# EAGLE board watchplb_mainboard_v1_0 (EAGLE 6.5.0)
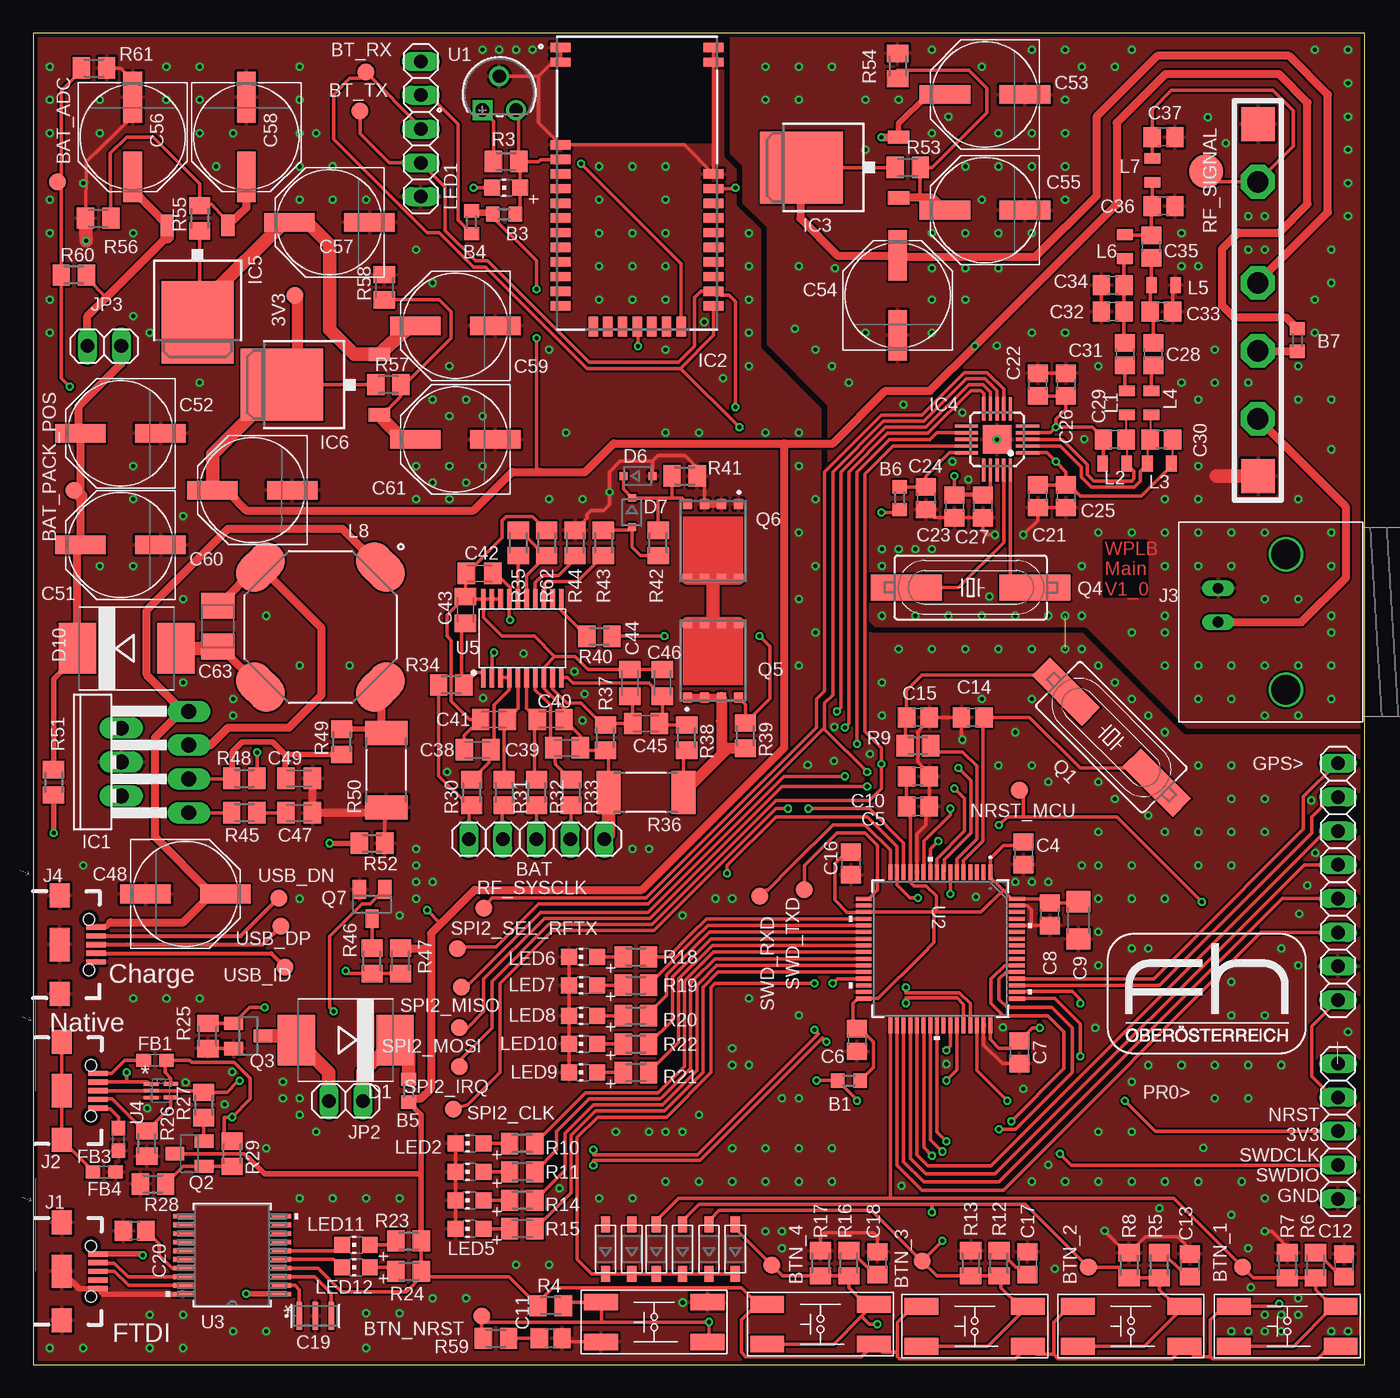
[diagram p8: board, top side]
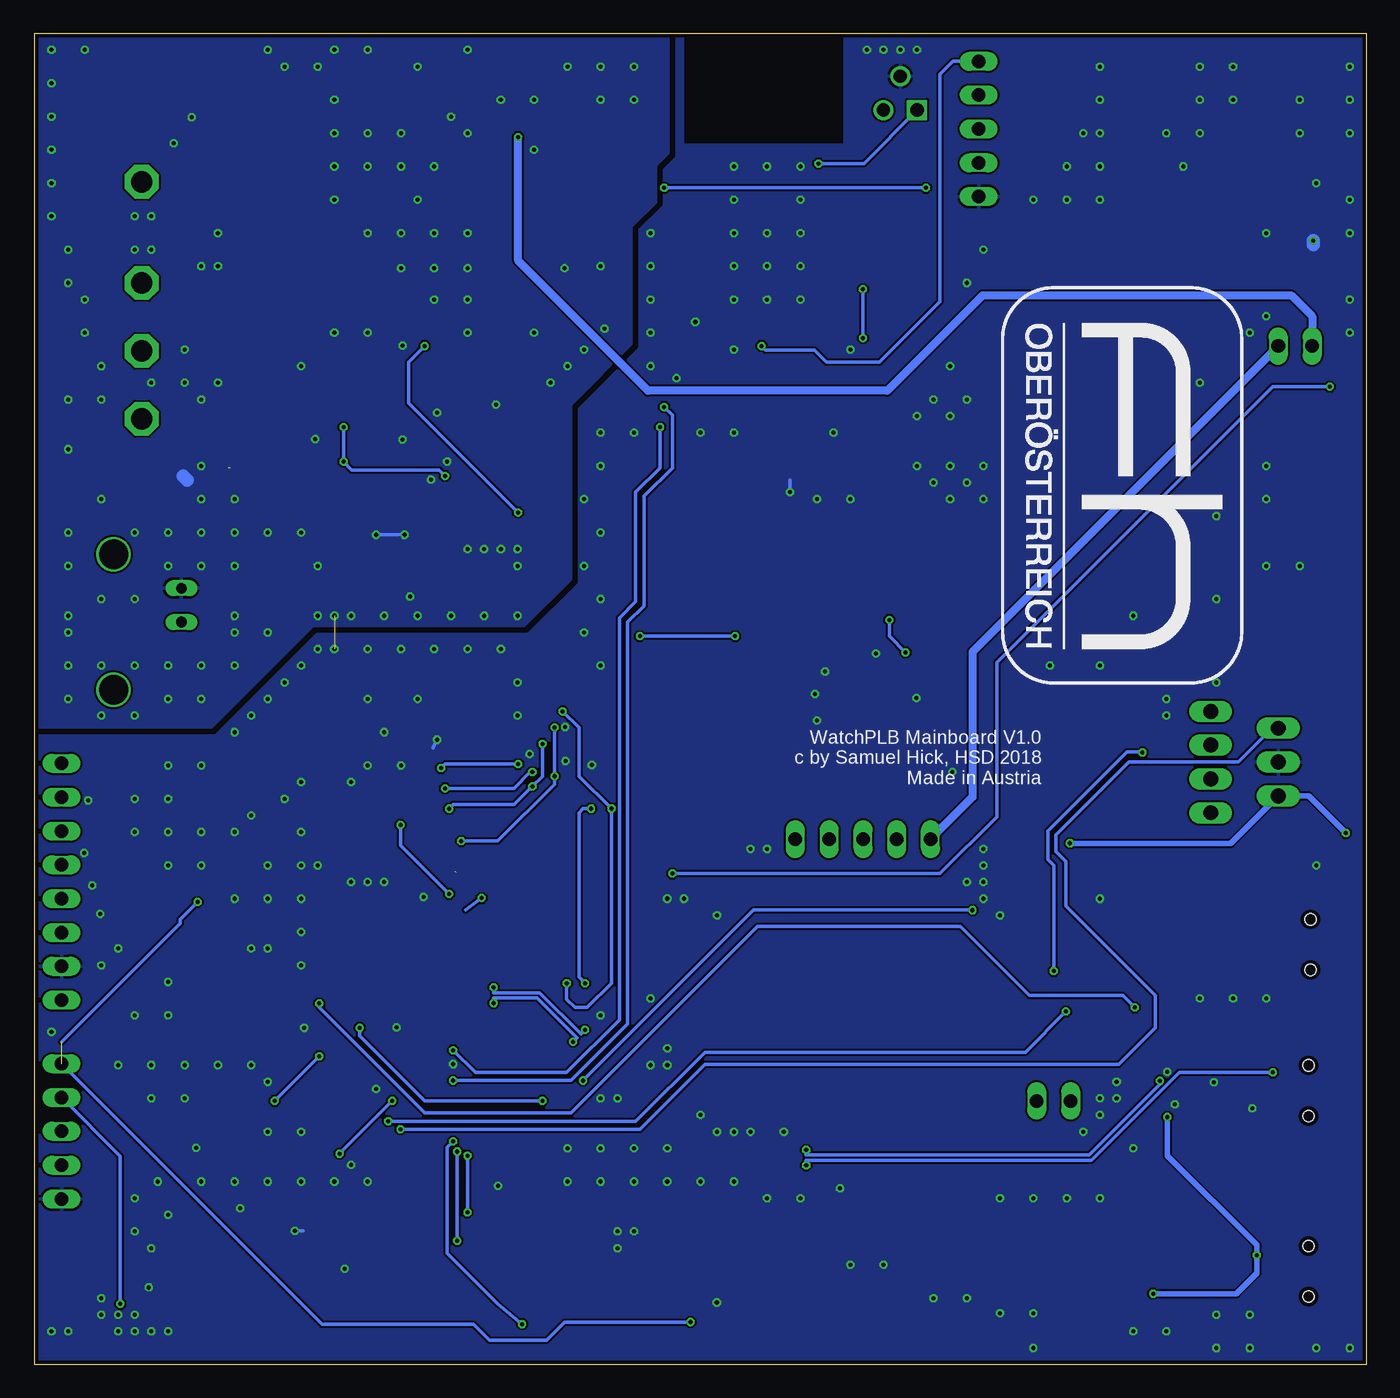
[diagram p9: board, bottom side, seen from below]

Size 100 x 100 mm. Coordinates in mm from the lower left corner, seen from the top.
Outline: 0,0 100,0 100,100 0,100 0,0
Copper layers (1*16): Top 0.035mm / dielectric 1.5mm / Bottom 0.035mm
Design rules "PCB-POOL Standard": minimum track width 0.15mm, minimum drill 0.3mm, track to track 0.15mm, track to pad 0.15mm, pad to pad 0.15mm, via to via 0.15mm, smd to smd 0.15mm, copper to edge 0.3mm, drill to drill 0.2mm, minimum pad ring 0.2mm, minimum via ring 0.15mm, stop-mask expansion 0.075mm, vias tented up to drill 0mil, thermal gap 0.2mm
tRestrict: area 39.3,91.7 to 51.2,99.7; 11 lines
bRestrict: area 39.3,91.7 to 51.2,99.7; 11 lines

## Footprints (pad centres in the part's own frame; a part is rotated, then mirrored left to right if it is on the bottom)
B1,27 = smd 1.27 x 1.27: TP 0,0
L0603 = smd 1 x 1.1: 1 -0.85,0; 2 0.85,0
1X05 = drill 1.016 long: 1 -5.08,0; 2 -2.54,0; 3 0,0; 4 2.54,0; 5 5.08,0
C0805 = smd 1.3 x 1.5: 1 -0.85,0; 2 0.85,0
C1206 = smd 1.6 x 1.8: 1 -1.4,0; 2 1.4,0
CSTCE = smd 0.406 x 2.108: 1 -1.2,0; 2 0,0; 3 1.2,0
C0805K = smd 1.3 x 1.6: 1 -1,0; 2 1,0
PANASONIC_E = smd 3.8 x 1.4: + 3,0; - -3,0
B/3528-21R = smd 1.95 x 2.5: + 1.525,0; - -1.525,0
SMC = smd 2.8 x 3.8: A 3.7,0; C -3.7,0
SOD-123 = smd 1.2 x 0.7: A 1.85,0; C -1.85,0
SOD323-R = smd 0.6 x 0.6: A 1.1,0; C -1.1,0
0603 = smd 1.1 x 1: 1 -0.85,0; 2 0.85,0
1X08 = drill 1.016 long: 1 -8.89,0; 2 -6.35,0; 3 -3.81,0; 4 -1.27,0; 5 1.27,0; 6 3.81,0; 7 6.35,0; 8 8.89,0
TO220-7 = drill 1.118 pad 1.626 long: 1 -3.81,-8.636; 2 -2.54,-3.556; 3 -1.27,-8.636; 4 0,-3.556; 5 1.27,-8.636; 6 2.54,-3.556; 7 3.81,-8.636
BM78SPPS5NC2_1 = smd 1.5 x 0.7: 1 -11.75,21.2; 2 -11.75,20.1; 3 -11.75,13.9; 4 -11.75,12.8; 5 -11.75,11.7; 6 -11.75,10.6; 7 -11.75,9.5; 8 -11.75,8.4; 9 -11.75,7.3; 10 -11.75,6.2; 11 -11.75,5.1; 12 -11.75,4; 13 -11.75,2.9; 14 -11.75,1.8; 22 -0.25,1.8; 23 -0.25,2.9; 24 -0.25,4; 25 -0.25,5.1; 26 -0.25,6.2; 27 -0.25,7.3; 28 -0.25,8.4; 29 -0.25,9.5; 30 -0.25,10.6; 31 -0.25,11.7; 32 -0.25,20.1; 33 -0.25,21.2 | smd 0.7 x 1.5: 15 -9.3,0.25; 16 -8.2,0.25; 17 -7.1,0.25; 18 -6,0.25; 19 -4.9,0.25; 20 -3.8,0.25; 21 -2.7,0.25
TO252 = smd 1 x 1.6: 1 -2.28,-4.8; 2 2.28,-4.8 | smd 5.4 x 6.2: TAB 0,2.5
QFN20 = smd 0.25 x 1.75: 1 -1,-2.3; 2 -0.5,-2.3; 3 0,-2.3; 4 0.5,-2.3; 5 1,-2.3; 11 1,2.3; 12 0.5,2.3; 13 0,2.3; 14 -0.5,2.3; 15 -1,2.3 | smd 1.75 x 0.25: 6 2.3,-1; 7 2.3,-0.5; 8 2.3,0; 9 2.3,0.5; 10 2.3,1; 16 -2.3,1; 17 -2.3,0.5; 18 -2.3,0; 19 -2.3,-0.5; 20 -2.3,-1 | smd 2.15 x 2.15: PAD 0,0
USB-B-MICRO-SMD = smd 1.45 x 0.4: D+ 2.725,0; D- 2.725,0.65; GND 2.725,-1.3; ID 2.725,-0.65; VBUS 2.725,1.3 | smd 1.5 x 1.8: SHIELD1 0,3.685; SHIELD2 0,-3.685 | smd 1.5 x 2.5: SHIELD3 0,0 | hole 0.85: 2.2,1.9; 2.2,-1.9
BNC = drill 2.2: 3 -5.08,5.08; 4 5.08,5.08 | drill 0.8 long: GND -2.54,0; S 0,0
1X02 = drill 1.016 long: 1 -1.27,0; 2 1.27,0
0805 = smd 0.8 x 1.2: 1 -0.9,0; 2 0.9,0
INDM115115X635N = smd 2.769 x 4.064: 1 -6.375,0; 3 6.375,0 | smd 4.064 x 2.769: 2 0,-6.375; 4 0,6.375
CHIP-LED0805 = smd 1.2 x 1.2: A 0,-1.05; C 0,1.05
HC49UP = smd 5.334 x 1.93: 1 -4.826,0; 2 4.826,0
SOT23-BEC = smd 1 x 1.4: B -0.95,-1.1; C 0,1.1; E 0.95,-1.1
SOT23 = smd 1 x 1.4: 1 -0.95,-1.1; 2 0.95,-1.1; 3 0,1.1
TRANS_CSD18534Q5A = smd 0.75 x 0.68: 1 -2.77,1.905; 2 -2.77,0.635; 3 -2.77,-0.635; 4 -2.77,-1.905 | smd 0.66 x 0.68: 5 2.78,-1.905; 6 2.78,-0.635; 7 2.78,0.635; 8 2.78,1.905
M0805 = smd 1.3 x 1.6: 1 -0.95,0; 2 0.95,0
R2512 = smd 1.8 x 3.2: 1 -2.8,0; 2 2.8,0
B2,54 = smd 2.54 x 2.54: TP 0,0
SMD_SWITCH = smd 2.54 x 1.27: P$1 4,1.5; P$2 -4,-1.5; P$3 -4,1.5; P$4 4,-1.5
TO-92_MC = drill 0.991 pad 1.499 square: 1 -2.54,-2.54 | drill 0.991 pad 1.499: 2 -1.27,0; 3 0,-2.54
LQFP64-10X10MM = smd 1.194 x 0.305: 1 -5.75,3.75; 2 -5.75,3.25; 3 -5.75,2.75; 4 -5.75,2.25; 5 -5.75,1.75; 6 -5.75,1.25; 7 -5.75,0.75; 8 -5.75,0.25; 9 -5.75,-0.25; 10 -5.75,-0.75; 11 -5.75,-1.25; 12 -5.75,-1.75; 13 -5.75,-2.25; 14 -5.75,-2.75; 15 -5.75,-3.25; 16 -5.75,-3.75; 33 5.75,-3.75; 34 5.75,-3.25; 35 5.75,-2.75; 36 5.75,-2.25; 37 5.75,-1.75; 38 5.75,-1.25; 39 5.75,-0.75; 40 5.75,-0.25; 41 5.75,0.25; 42 5.75,0.75; 43 5.75,1.25; 44 5.75,1.75; 45 5.75,2.25; 46 5.75,2.75; 47 5.75,3.25; 48 5.75,3.75 | smd 0.305 x 1.194: 17 -3.75,-5.75; 18 -3.25,-5.75; 19 -2.75,-5.75; 20 -2.25,-5.75; 21 -1.75,-5.75; 22 -1.25,-5.75; 23 -0.75,-5.75; 24 -0.25,-5.75; 25 0.25,-5.75; 26 0.75,-5.75; 27 1.25,-5.75; 28 1.75,-5.75; 29 2.25,-5.75; 30 2.75,-5.75; 31 3.25,-5.75; 32 3.75,-5.75; 49 3.75,5.75; 50 3.25,5.75; 51 2.75,5.75; 52 2.25,5.75; 53 1.75,5.75; 54 1.25,5.75; 55 0.75,5.75; 56 0.25,5.75; 57 -0.25,5.75; 58 -0.75,5.75; 59 -1.25,5.75; 60 -1.75,5.75; 61 -2.25,5.75; 62 -2.75,5.75; 63 -3.25,5.75; 64 -3.75,5.75
SSOP20_MC = smd 1.473 x 0.356: 1 -3.708,2.926; 2 -3.708,2.276; 3 -3.708,1.626; 4 -3.708,0.975; 5 -3.708,0.325; 6 -3.708,-0.325; 7 -3.708,-0.975; 8 -3.708,-1.626; 9 -3.708,-2.276; 10 -3.708,-2.926; 11 3.708,-2.926; 12 3.708,-2.276; 13 3.708,-1.626; 14 3.708,-0.975; 15 3.708,-0.325; 16 3.708,0.325; 17 3.708,0.975; 18 3.708,1.626; 19 3.708,2.276; 20 3.708,2.926
SOT50P160X60-5N = smd 1.118 x 0.254: 1 -0.737,0.508; 2 -0.737,0; 3 -0.737,-0.508 | smd 1.118 x 0.305: 4 0.737,-0.508; 5 0.737,0.508
TSSOP-20/6MM = smd 1.5 x 0.35: 1 -2.95,2.925; 2 -2.95,2.275; 3 -2.95,1.625; 4 -2.95,0.975; 5 -2.95,0.325; 6 -2.95,-0.325; 7 -2.95,-0.975; 8 -2.95,-1.625; 9 -2.95,-2.275; 10 -2.95,-2.925; 11 2.95,-2.925; 12 2.95,-2.275; 13 2.95,-1.625; 14 2.95,-0.975; 15 2.95,-0.325; 16 2.95,0.325; 17 2.95,0.975; 18 2.95,1.625; 19 2.95,2.275; 20 2.95,2.925
RA07H4047M = drill 1.6 pad 2.54 octagon: 1 6.1,1.75; 2 13.7,1.75; 3 18.8,1.75; 4 23.9,1.75 | smd 2.54 x 2.54: 5_L 1.778,1.778; 5_R 28.194,1.778

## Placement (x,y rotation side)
3V3  PTR1B1,27  [B1,27]  19.66,80.31 90 top
B1  BLM18KG601SN1D  [L0603]  61.26,21.34 0 top
B3  BLM18KG601SN1D  [L0603]  35.36,86.41 0 top
B4  BLM18KG601SN1D  [L0603]  32.92,85.8 270 top
B5  BLM18KG601SN1D  [L0603]  28.19,20.57 90 top
B6  BLM18KG601SN1D  [L0603]  65.07,65.07 90 top
B7  BLM18KG601SN1D  [L0603]  94.95,76.96 270 top
BAT  [1X05]  37.8,39.47 0 top
BAT_ADC  PTR1B1,27  [B1,27]  1.83,88.85 0 top
BAT_PACK_POS  PTR1B1,27  [B1,27]  3.05,65.68 0 top
BT_RX  PTR1B1,27  [B1,27]  24.99,97.08 0 top
BT_TX  PTR1B1,27  [B1,27]  24.54,94.18 0 top
BTN_1  PTR1B1,27  [B1,27]  90.83,7.32 180 top
BTN_2  PTR1B1,27  [B1,27]  79.25,7.32 180 top
BTN_3  PTR1B1,27  [B1,27]  66.75,7.77 180 top
BTN_4  PTR1B1,27  [B1,27]  55.47,7.47 180 top
BTN_NRST  PTR1B1,27  [B1,27]  33.68,3.66 180 top
C4  100nF  [C0805]  74.37,38.4 270 top
C5  100nF  [C0805]  66.45,41.91 180 top
C6  100nF  [C0805]  61.87,24.38 90 top
C7  100nF  [C0805]  74.07,23.47 270 top
C8  100nF  [C0805]  76.35,33.83 270 top
C9  10uF  [C1206]  78.49,33.38 270 top
C10  1uF  [C0805]  66.45,44.2 180 top
C11  100nF  [C0805]  38.86,1.98 180 top
C12  100nF  [C0805]  98.45,7.47 270 top
C13  100nF  [C0805]  86.87,7.47 270 top
C14  27p  [C0805]  70.56,48.62 180 top
C15  27p  [C0805]  66.45,48.62 0 top
C16  100nF  [C0805]  61.42,37.64 90 top
C17  100nF  [C0805]  74.68,7.62 270 top
C18  100nF  [C0805]  63.4,7.62 270 top
C19  CSTCE12M0G15L99-R0  [CSTCE]  21.18,3.66 0 top
C20  1uF  [C0805]  7.62,10.06 180 top
C21  100nF  [C0805]  75.44,65.23 90 top
C22  100nF  [C0805]  75.44,73.61 270 top
C23  100nF  [C0805]  69.19,64.47 90 top
C24  100nF  [C0805]  67.06,65.07 90 top
C25  27pF  [C0805]  77.57,65.23 90 top
C26  27pF  [C0805]  77.57,73.61 270 top
C27  1uF  [C0805]  71.32,64.47 90 top
C28  [C0805]  84.12,75.9 90 top
C29  [C0805]  81.23,69.49 180 top
C30  [C0805]  84.73,69.49 180 top
C31  [C0805]  81.99,75.9 90 top
C32  [C0805]  81.08,79.1 0 top
C33  [C0805]  84.73,79.1 0 top
C34  [C0805]  81.08,81.08 0 top
C35  [C0805]  83.97,83.97 270 top
C36  [C0805]  84.89,87.02 180 top
C37  [C0805]  84.89,92.2 180 top
C38  100nF  [C0805K]  33.38,46.18 180 top
C39  100nF  [C0805K]  40.08,46.33 0 top
C40  100nF  [C0805K]  38.86,48.46 0 top
C41  100nF  [C0805K]  34.59,48.46 180 top
C42  1uF  [C0805K]  33.53,59.44 0 top
C43  1uF  [C0805K]  32.46,56.69 90 top
C44  100nF  [C0805K]  44.81,51.21 270 top
C45  100nF  [C0805K]  46.02,48.16 0 top
C46  100nF  [C0805K]  47.24,51.21 90 top
C47  100nF  [C0805K]  19.96,41.45 180 top
C48  22uF 80-EDK226M050A9GAA  [PANASONIC_E]  11.43,35.36 0 top
C49  100nF  [C0805K]  19.96,44.04 180 top
C51  22uF 80-EDK226M050A9GAA  [PANASONIC_E]  6.55,61.57 180 top
C52  22uF 80-EDK226M050A9GAA  [PANASONIC_E]  6.55,69.95 180 top
C53  10uF 80-EDK106M025A9DAA  [PANASONIC_E]  71.48,95.4 180 top
C54  100uF 647-GYA1E101MCQ1GS  [PANASONIC_E]  64.92,80.31 90 top
C55  NP  [PANASONIC_E]  71.48,86.72 180 top
C56  10uF 80-EDK106M025A9DAA  [PANASONIC_E]  7.47,92.2 270 top
C57  100uF 647-GYA1E101MCQ1GS  [PANASONIC_E]  22.25,85.8 180 top
C58  NP  [PANASONIC_E]  16,92.2 270 top
C59  10uF 80-EDK106M025A9DAA  [PANASONIC_E]  31.7,78.03 180 top
C60  100uF 647-GYA1E101MCQ1GS  [PANASONIC_E]  16.46,65.68 180 top
C61  NP  [PANASONIC_E]  31.7,69.49 180 top
C63  4.7uF low esr 80-T521B475M35ATE150  [B/3528-21R]  13.87,55.47 90 top
CONFIG_INTERFACE_TEST_POINT  [1X05]  29.11,92.81 270 top
D1  S8NC-13  [SMC]  23.47,24.38 180 top
D2  [SOD-123]  46.79,8.69 90 top
D3  [SOD-123]  48.77,8.69 90 top
D4  [SOD-123]  50.75,8.69 90 top
D5  [SOD-123]  52.73,8.69 90 top
D6  Zener 16V MMSZ5246BS-7-F  [SOD323-R]  45.42,66.75 0 top
D7  100V, BAS16J,135  [SOD323-R]  44.96,64.01 270 top
D8  [SOD-123]  44.96,8.69 90 top
D9  [SOD-123]  42.98,8.69 90 top
D10  MBRS330T3  [SMC]  7.01,53.8 0 top
FB1  BLM18PG300SN1D  [0603]  9.14,22.86 0 top
FB3  BLM18PG300SN1D  [0603]  6.4,16.92 90 top
FB4  BLM18PG300SN1D  [0603]  5.33,14.48 180 top
GPS>  [1X08]  97.99,36.27 90 top
IC1  LT1513  [TO220-7]  3.05,45.26 90 top
IC2  BM70BLES1FC2-0B03AA  [BM78SPPS5NC2_1]  51.36,77.72 0 top
IC3  LM1117DTX-ADJ-12V  [TO252]  60.2,89.92 90 top
IC4  AX5031  [QFN20]  72.39,69.49 90 top
IC5  LM1117DTX-ADJ-10V  [TO252]  12.34,80.77 180 top
IC6  LM1117DTX-ADJ-3V3  [TO252]  21.18,73.61 90 top
J1  [USB-B-MICRO-SMD]  2.13,7.01 0 top
J2  [USB-B-MICRO-SMD]  2.13,20.57 0 top
J3  BNCPTH  [BNC]  89,55.78 270 top
J4  [USB-B-MICRO-SMD]  1.98,31.55 0 top
JP2  VIB_MOTOR, 619-28821  [1X02]  23.47,19.81 180 top
JP3  Power Disconnect  [1X02]  5.33,76.5 180 top
L1  [0805]  82.14,72.24 270 top
L2  [0805]  81.23,67.67 0 top
L3  [0805]  84.58,67.67 0 top
L4  [0805]  83.97,72.24 270 top
L5  [0805]  84.89,81.08 180 top
L6  [0805]  81.99,83.97 90 top
L7  [0805]  84.05,89.69 90 top
L8  CTX10-4A-R  [INDM115115X635N]  21.57,55.4 225 top
LED1  BLUE  [CHIP-LED0805]  35.51,88.39 90 top
LED2  GREEN  [CHIP-LED0805]  32.77,16.61 90 top
LED3  BLUE  [CHIP-LED0805]  32.77,14.48 90 top
LED4  WHITE  [CHIP-LED0805]  32.77,12.34 90 top
LED5  RED  [CHIP-LED0805]  32.77,10.21 90 top
LED6  GREEN  [CHIP-LED0805]  41.3,30.63 90 top
LED7  GREEN  [CHIP-LED0805]  41.3,28.5 90 top
LED8  GREEN  [CHIP-LED0805]  41.3,26.21 90 top
LED9  RED  [CHIP-LED0805]  41.3,21.95 90 top
LED10  YELLOW  [CHIP-LED0805]  41.3,24.08 90 top
LED11  GREEN  [CHIP-LED0805]  24.23,8.99 90 top
LED12  RED  [CHIP-LED0805]  24.23,7.32 90 top
NRST_MCU  PTR1B1,27  [B1,27]  74.07,43.13 180 top
PR0>  SWD  [1X05]  97.99,17.53 90 top
Q1  8MHz / LFXTAL020423Reel  [HC49UP]  80.97,47.14 315 top
Q2  BC817-25SMD  [SOT23-BEC]  11.73,15.85 90 top
Q3  DMN3023L-7  [SOT23]  16.15,24.69 270 top
Q4  16MHz_LFXTAL051370Reel  [HC49UP]  70.41,58.37 180 top
Q5  CSD18534Q5A  [TRANS_CSD18534Q5A]  51.05,52.88 90 top
Q6  CSD18534Q5A  [TRANS_CSD18534Q5A]  51.05,61.87 270 top
Q7  DMN3023L-7  [SOT23]  25.45,34.59 180 top
R3  4k7  [M0805]  35.51,90.37 180 top
R4  47k  [M0805]  38.86,4.42 0 top
R5  10k  [M0805]  84.58,7.47 270 top
R6  10k  [M0805]  96.32,7.47 270 top
R7  10k  [M0805]  94.18,7.47 90 top
R8  10k  [M0805]  82.3,7.47 90 top
R9  220R  [M0805]  66.45,46.48 0 top
R10  470R  [M0805]  36.73,16.61 0 top
R11  470R  [M0805]  36.73,14.48 0 top
R12  10k  [M0805]  72.54,7.62 270 top
R13  10k  [M0805]  70.41,7.62 90 top
R14  470R  [M0805]  36.73,12.34 0 top
R15  470R  [M0805]  36.73,10.21 0 top
R16  10k  [M0805]  61.26,7.62 270 top
R17  10k  [M0805]  59.13,7.62 90 top
R18  470R  [M0805]  45.26,30.63 180 top
R19  470R  [M0805]  45.26,28.5 180 top
R20  470R  [M0805]  45.26,26.21 180 top
R21  470R  [M0805]  45.26,21.95 180 top
R22  470R  [M0805]  45.26,24.08 180 top
R23  220R  [M0805]  28.19,9.3 180 top
R24  220R  [M0805]  28.19,7.01 180 top
R25  100k  [M0805]  13.11,24.69 270 top
R26  100k  [M0805]  8.53,16.61 270 top
R27  x  [M0805]  12.8,19.51 90 top
R28  x  [M0805]  8.99,13.56 180 top
R29  x  [M0805]  14.94,15.85 270 top
R30  1k  [M0805]  32.92,42.98 90 top
R31  1k  [M0805]  35.36,42.98 90 top
R32  1k  [M0805]  37.8,42.98 90 top
R33  1k  [M0805]  40.39,42.98 90 top
R34  1k  [M0805]  31.39,51.05 0 top
R35  10k  [M0805]  36.42,61.72 90 top
R36  20mR  [R2512]  46.02,42.98 180 top
R37  100R  [M0805]  42.98,47.09 270 top
R38  100R  [M0805]  49.07,47.09 270 top
R39  10M  [M0805]  53.49,47.24 270 top
R40  5k1  [M0805]  42.52,54.71 180 top
R41  3M3  [M0805]  48.92,66.75 180 top
R42  1M  [M0805]  46.94,61.72 270 top
R43  5k1  [M0805]  42.82,61.72 90 top
R44  470k  [M0805]  40.69,61.72 90 top
R45  330  [M0805]  15.85,41.45 0 top
R46  910R  [M0805]  25.45,30.33 270 top
R47  10k  [M0805]  27.58,30.33 270 top
R48  330k  [M0805]  15.85,44.04 180 top
R49  10k  [M0805]  23.16,46.79 90 top
R50  0.25R  [R2512]  26.52,44.65 90 top
R51  120k  [M0805]  1.52,43.74 90 top
R52  12k4  [M0805]  25.45,39.17 180 top
R53  5k1  [M0805]  65.68,89.92 0 top
R54  47k  [M0805]  64.92,97.54 90 top
R55  5k1  [M0805]  12.5,86.11 90 top
R56  47k  [M0805]  4.88,86.11 180 top
R57  5k1  [M0805]  26.67,73.61 0 top
R58  47k  [M0805]  26.37,80.92 90 top
R59  10k  [M0805]  34.75,1.98 180 top
R60  47k  [M0805]  3.05,81.84 0 top
R61  10k  [M0805]  4.57,97.38 180 top
R62  NTC 103AT  [M0805]  38.56,61.72 90 top
RF_SIGNAL  PTR1B2,54  [B2,54]  88.09,89.61 0 top
RF_SYSCLK  PTR1B1,27  [B1,27]  33.83,34.29 180 top
S1  [SMD_SWITCH]  46.63,3.2 180 top
S2  [SMD_SWITCH]  94.18,2.9 180 top
S3  [SMD_SWITCH]  82.45,2.9 180 top
S4  [SMD_SWITCH]  70.71,2.9 180 top
S5  [SMD_SWITCH]  59.13,3.05 180 top
SPI2_CLK  PTR1B1,27  [B1,27]  31.55,19.2 180 top
SPI2_IRQ  PTR1B1,27  [B1,27]  32,22.4 180 top
SPI2_MISO  PTR1B1,27  [B1,27]  32.16,28.35 180 top
SPI2_MOSI  PTR1B1,27  [B1,27]  32,25.3 180 top
SPI2_SEL_RFTX  PTR1B1,27  [B1,27]  31.85,31.24 180 top
SWD_RXD  PTR1B1,27  [B1,27]  54.56,35.2 180 top
SWD_TXD  PTR1B1,27  [B1,27]  57.91,35.66 180 top
U1  MCP111-XXXXX/TO  [TO-92_MC]  36.27,96.77 0 top
U2  STM32L073RZ  [LQFP64-10X10MM]  68.12,31.24 270 top
U3  MCP2200-I/SS  [SSOP20_MC]  14.94,8.23 180 top
U4  TPD3E001DRLR  [SOT50P160X60-5N]  9.6,20.57 0 top
U5  BQ7790504  [TSSOP-20/6MM]  36.73,54.56 90 top
U$2  RA07H4047M  [RA07H4047M]  90.22,94.95 270 top
U$4  [FH_LOGO]  27.74,81.38 270 bottom
U$5  [FH_LOGO_050]  80.47,23.16 0 top
USB_DN  PTR1B1,27  [B1,27]  18.44,35.05 90 top
USB_DP  PTR1B1,27  [B1,27]  18.59,32.92 90 top
USB_ID  PTR1B1,27  [B1,27]  18.9,29.87 90 top

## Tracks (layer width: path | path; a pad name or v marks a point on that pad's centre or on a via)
10V_INTERMEDIATE
  Top 0.254: R55.1 12.5,78.33 IC5.TAB
  Top 0.813: C57.+ 19.4,85.65 20.73,85.65
  Top 1.016: C57.+ 18.9,85.8 13.11,80.16 13.11,78.94 IC5.TAB | C59.+ 28.35,78.03 IC6.2 24.09,75.89 22.25,77.72 22.25,84.12 20.73,85.65
+3V3  (via drill 0.3)
  Top 0.254: R57.1 19.81,73.61 IC6.TAB | 97.71,1.4 S2.P$3 98.01,1.22 97.23,1.22 96.47,0.46 88.54,0.46 88.39,0.61 | 88.39,0.61 88.39,3.35 89.31,4.27 90.06,4.27 S2.P$4 93.4,4.4 v93.57,4.57 | 76.66,0.76 76.66,3.2 77.85,4.4 S3.P$4 78.02,3.96 77.42,3.96 | S4.P$4 66.12,4.4 64.92,3.2 64.92,0.91 | 54.1,4.27 53.19,3.35 53.19,0.91 53.49,0.61 62.19,0.61 S5.P$3 63.77,0.91 64.92,0.91 | S5.P$4 54.85,4.27 54.1,4.27 | 76.66,0.76 76.96,0.46 85.51,0.46 S3.P$3 87.23,0.61 88.39,0.61 | 76.66,0.76 75.35,0.76 S4.P$3 73.78,0.46 65.08,0.46 64.92,0.61 64.92,0.91 | 54.1,4.27 54.41,4.57 | Q2.C 15.85,15.85 16.15,15.54 | B6.1 64.86,64.01 v63.7,64.01 | B3.1 33.16,86.41 B4.1 34.05,86.65 37.8,82.91 v37.8,80.77 | R23.1 R24.1 29.14,6.59 | U3.4 21.4,7.25 23.16,5.49 28.04,5.49 29.14,6.59 | 29.14,6.59 35.74,6.59 R4.1 37.91,4.69 39.01,5.79 53.19,5.79 54.41,4.57 | v29.57,34.14 30.6,33.11 | v61.87,19.81 61.57,20.18 B1.1 v58.83,21.34 | v37.8,77.11 37.8,67.36 38.1,67.06 | v75.59,25.3 75.05,25.3 C7.1 74,24.32 73.46,23.77 72.54,23.77 71.87,24.44 U2.48 | GPS>.1 96.01,25.4 96.01,21.64 97.59,20.07 PR0>.4 | 54.86,4.57 54.41,4.57
  Top 0.406: B5.1 29.14,18.77 29.14,14.33 | 29.14,14.33 R23.1 | 16.15,15.54 17.37,14.33 29.14,14.33
  Top 0.61: B7.1 94.12,78.64 90.22,78.64 89.31,79.55 89.31,83.82 90.53,85.04 93.57,85.04 95.71,87.17 95.71,94.79 93.57,96.93 85.04,96.93 81.38,93.27 81.38,87.17 v70.71,76.5 | v70.71,76.5 70.41,76.2 | C60.+ 13.61,65.53 14.63,65.53 16,64.16 33.07,64.16 35.97,67.06 38.1,67.06 41.45,67.06 43.59,69.19 56.39,69.19 | v70.71,76.5 67.36,73.15 64.01,73.15 60.05,69.19 56.39,69.19 | 56.39,69.19 56.39,46.33 45.72,35.66 33.15,35.66 30.6,33.11 29.87,32.38 29.87,31.24 | 29.87,31.24 29.87,20.73 29.11,19.96 28.65,19.96 28.41,19.72 B5.1 | R47.1 29.84,31.28 29.87,31.24
  Top 0.813: 3V3.TP 19.81,80.16 19.81,73.61
  Top 1.016: C60.+ 13.46,68.39 IC6.TAB
  Bottom 0.254: v63.7,64.01 71.93,72.24 71.93,75.29 v70.71,76.5 | v29.57,34.14 46.02,34.14 v58.83,21.34 | v61.87,19.81 70.71,19.81 75.59,24.69 v75.59,25.3 | v37.8,80.77 v37.8,77.11 | v93.57,4.57 93.57,15.65 PR0>.4
+5V  (via drill 0.3)
  Top 0.254: R29.1 14.33,17.41 14.33,18.59 v14.94,18.59 16.31,19.96 16.31,21.49 15.09,22.71 11.89,22.71 11.73,22.86 FB1.2 9.91,22.77 9.91,21.95 10.34,21.51 U4.5 | U3.1 18.61,5.33
  Top 0.406: 18.61,5.33 v16,5.33 | v8.23,8.23 8.15,8.31 J1.VBUS
  Bottom 0.406: v14.94,18.59 14.94,15.7 8.23,8.99 v8.23,8.23 8.23,6.86 9.75,5.33 v16,5.33
+12V
  Top 0.254: R53.1 IC3.TAB
  Top 0.61: 64.92,83.36 C54.+ 60.4,83.31 57.61,86.11 57.61,87.33 59.59,89.31 | 91.97,81.3 97.23,86.56 97.23,95.4 94.34,98.3 84.43,98.3 79.86,93.73 79.86,87.78 75.29,83.21 65.08,83.21 64.92,83.36 | 64.92,83.97 64.92,83.36
  Top 1.016: 59.59,89.31 58.37,89.31 IC3.TAB | U$2.2 91.97,81.3
ANT_N
  Top 0.15: L1.2 82.08,71.27 C29.1 82.13,69.44 L2.2
  Top 0.254: IC4.3 77.28,69.49 79.17,67.61 79.17,66.85 79.65,66.37 82.51,66.37 82.68,66.54 82.68,67.12 L2.2
ANT_P
  Top 0.15: L4.2 83.88,71.25 C30.2 83.68,69.29 L3.1
  Top 0.254: IC4.2 77.14,68.99 78.72,67.42 78.72,66.66 79.46,65.91 82.69,65.91 83.13,66.35 83.13,67.12 L3.1
BAT_ADC  (via drill 0.3)
  Top 0.254: 2.1,89 R60.1 2.1,74.1 v2.74,73.46 | 2.1,89 2.1,95.67 3.35,96.93 3.35,97.11 R61.2 | BAT_ADC.TP 1.95,88.85 2.1,89 | v66.45,35.05 65.84,35.05 64.87,36.02 U2.15 64.87,38.91 62.64,41.15 55.78,41.15 52.12,37.49 v52.12,36.88
  Bottom 0.254: v66.45,35.05 67.67,34.14 | v2.74,73.46 7.01,73.46 27.74,52.73 27.74,41.15 32,36.88 v52.12,36.88
BAT_PACK_GND
  Top 0.254: 32.16,46.18 C38.2 32.38,47.24 C41.2 32.77,48.46 31.39,49.84 31.39,54.41 31.09,54.71 31.09,56.32 C43.2 | U5.20 U5.19 U5.18 | R36.2 43.23,45.89 R37.2 41.27,46.14 C39.2 41.08,47.24 C40.2 39.93,48.53 39.93,49.23 38.35,50.8 U5.8 38.35,52.37 39.17,53.19 | C46.2 C44.1 41.67,52.21 40.69,53.19 39.17,53.19 | R62.2 38.56,62.94 38.25,62.94 37.49,63.7 35.51,63.7 35.2,63.4 35.2,62.11 C42.1 32.46,59.37 C43.2 | U5.20 32.65,57.51 C43.2 | 39.17,53.19 37.64,54.71 35.2,54.71 33.8,56.11 U5.20
  Top 1.016: R36.2 43.23,39.82 BAT.5
BAT_PACK_POS
  Top 0.254: BAT.1 32.72,41.82 R30.1 32.73,42.22 32.46,42.22 30.44,44.23 R34.1
  Top 0.406: R51.2 1.52,51.51 3.05,53.03 3.05,53.53 D10.C
  Top 0.61: D10.C 3.31,61.33 | C51.+ 3.55,65.23 C52.+ | 3.4,70.15 3.4,71.98 6.6,75.18 JP3.1
  Top 1.016: 3.31,61.33 C51.+ | C52.+ 3.4,70.1 | 3.4,70.1 2.13,70.1 | 3.4,70.1 3.4,70.15 | BAT_PACK_POS.TP 3.1,65.68 3.55,65.23
  Bottom 0.61: BAT.1 29.57,42.62 29.57,53.54 JP3.1
BT_HCI_RXD  (via drill 0.3)
  Top 0.254: IC2.22 51.11,77.32 48.62,74.83 | 48.62,74.83 41.6,74.83 33.98,82.45 33.07,82.45 30.48,85.04 29.57,85.04 22.55,92.05 22.55,95.4 23.77,96.62 24.54,96.62 BT_RX.TP 29.11,92.96 CONFIG_INTERFACE_TEST_POINT.3 | 48.62,74.83 v53.03,70.41 | U2.42 68.89,25.48 68.89,23.93 v68.58,23.62
  Bottom 0.254: v53.03,70.41 53.03,67.36 54.86,65.53 54.86,57.3 56.08,56.08 56.08,25.91 60.05,21.95 66.9,21.95 v68.58,23.62
BT_HCI_TXD  (via drill 0.3)
  Top 0.254: v52.73,71.93 52.73,79.86 52.27,80.31 51.66,80.31 51.35,80.62 IC2.23 50.14,80.62 49.68,80.16 49.68,76.5 48.46,75.29 41.76,75.29 34.14,82.91 33.22,82.91 30.94,85.19 30.94,88.44 CONFIG_INTERFACE_TEST_POINT.4 26.72,90.27 24.54,92.46 BT_TX.TP | U2.43 69.37,22.13 v68.58,21.34
  Bottom 0.254: v52.73,71.93 52.12,71.32 52.12,67.36 54.25,65.23 54.25,57 55.47,55.78 55.47,25.6 59.74,21.34 v68.58,21.34
BT_NRST  (via drill 0.3)
  Top 0.254: U1.1 34.56,93.41 R3.2 | IC2.21 48.66,82.71 v41.15,90.22
  Bottom 0.254: v41.15,90.22 37.74,90.22 U1.1
BT_P2_0_MODE  (via drill 0.3)
  Top 0.254: v45.41,76.5 45.41,77.92 IC2.18
  Bottom 0.254: CONFIG_INTERFACE_TEST_POINT.1 31.04,97.89 32,96.93 32,85.65 32,79.86 35.66,76.2 36.58,75.29 40.54,75.29 41.45,76.2 45.11,76.2 v45.41,76.5
BTN_1
  Top 0.254: S2.P$1 94.66,1.4 97.54,4.27 98.06,4.27 S2.P$2 97.85,4.72 97.23,4.72 96.32,5.64 R6.2 R7.1 91.63,6.52 BTN_1.TP 85.65,12.5 64.31,12.5 | D2.A 46.79,10.82 48.46,12.5 64.31,12.5 | U2.33 64.37,12.56 64.31,12.5
BTN_2  (via drill 0.3)
  Top 0.254: S3.P$1 83.45,1.4 S3.P$2 86.27,4.57 85.65,4.57 84.58,5.64 R5.2 R8.1 81.5,7.32 BTN_2.TP 74.52,12.04 67.51,12.04 | D3.A 48.77,10.82 49.99,12.04 67.51,12.04 | U2.38 66.9,25.46 66.9,16.31 v67.51,15.7 | v67.51,11.43 67.51,12.04
  Bottom 0.254: v67.51,15.7 v67.51,11.43
BTN_3  (via drill 0.3)
  Top 0.254: S4.P$1 71.71,1.4 S4.P$2 74.09,4.4 72.69,5.79 72.69,6.52 R12.2 R13.1 67.85,6.67 BTN_3.TP | 50.77,10.54 D4.A 50.9,10.69 50.9,10.97 51.51,11.58 62.94,11.58 BTN_3.TP | U2.39 67.37,16.9 v68.28,16 | v68.28,9.3 BTN_3.TP
  Bottom 0.254: v68.28,16 v68.28,9.3
BTN_4  (via drill 0.3)
  Top 0.254: 62.21,3.63 S5.P$2 62.95,4.72 62.33,4.72 61.27,5.79 R16.2 R17.1 56.27,6.67 BTN_4.TP 52.73,10.21 D5.A | 62.21,3.63 60.13,1.55 S5.P$1 | v63.4,3.05 62.79,3.05 62.21,3.63 | U2.40 67.87,17.47 v68.58,16.76
  Bottom 0.254: v63.4,3.05 65.23,4.57 69.04,8.38 69.04,16.31 v68.58,16.76
CHARGER_CH_PRECH  (via drill 0.3)
  Top 0.254: U2.54 72.97,29.99 71.93,28.96 71.93,27.13 72.85,26.21 76.2,26.21 77.42,24.99 77.42,22.25 v73.46,18.29 | v22.55,26.52 22.25,26.82 22.25,32.16 24.69,34.59 25.3,34.59 Q7.1
  Bottom 0.254: v73.46,18.29 54.86,18.29 49.68,23.47 25.6,23.47 v22.55,26.52
CHARGER_SS  (via drill 0.3)
  Top 0.254: U2.53 73.08,29.49 72.54,28.96 72.54,27.43 73.15,26.82 76.5,26.82 78.03,25.3 78.03,21.95 73.76,17.68 v72.54,17.68
  Bottom 0.254: IC1.6 7.06,47.8 9.6,45.26 17.83,45.26 23.32,39.78 23.32,38.56 22.55,37.8 22.55,34.44 15.85,27.74 15.85,25.3 18.59,22.55 49.68,22.55 54.56,17.68 v72.54,17.68
GND  (via drill 0.3)  (1 unrouted)
  Top 0.254: R56.2 3.96,90.37 7.47,93.73 C56.- 7.01,95.66 7.01,96.93 6.55,97.38 R61.1 | C59.- 33.38,78.03 | S1.P$1 39.99,1.7 C11.1 | C13.1 86.87,8.69 85.95,9.6 83.52,9.6 82.33,8.42 R8.2 82.11,8.42 v80.47,10.06 | R25.2 Q3.2 | Q6.3 50.42,66.2 R41.1 50.17,67.05 48.95,68.28 46.94,68.28 46.52,67.85 | R44.2 41.6,63.59 41.6,63.86 41.91,64.16 42.82,64.16 43.28,64.62 v43.28,65.53 43.28,67.06 44.08,67.85 46.52,67.85 | R52.1 26.4,41.17 26.12,41.45 | C26.1 C22.1 | v74.37,62.33 75.44,63.4 C21.1 C25.1 | 85.48,79.5 C33.2 85.58,80.87 L5.1 | C34.1 C32.1 | 46.52,67.85 D6.A | 26.36,81.84 R58.2 | U1.2 37.95,96.77 | 37.95,96.77 39.01,97.84 39.59,97.84 IC2.2 IC2.1 | 37.95,96.77 37.95,93.28 IC2.3 48.91,91.62 IC2.31 IC2.32 IC2.33 | 21.18,2.9 C19.2 | U2.60 74.98,32.99 | 74.98,32.99 76.34,32.99 C8.2 | U2.63 74.63,34.49 74.98,34.14 74.98,32.99 | C7.2 72.78,22.62 71.37,24.03 U2.47 | U2.12 66.37,39.85 67.06,40.54 67.06,41.06 C5.1 67.3,44.41 66.45,45.26 66.45,47.55 66.9,48.01 66.9,48.22 C15.2 C14.2 69.71,47.03 v69.8,46.94 | LED9.C LED10.C LED8.C LED7.C LED6.C | LED2.C LED3.C LED4.C LED5.C | R7.2 94.18,8.84 93.02,10 v92.5,10 | U4.3 8.48,20.07 | C18.1 63.4,9.6 63.09,9.91 59.44,9.91 59.13,9.6 R17.2 | C24.1 67.67,63.62 C23.1 C27.1 71.32,62.64 71.63,62.33 v72.24,62.33
  Top 0.406: J1.SHIELD3 3.43,5.71 J1.GND 5.26,5.3 U3.20
  Top 0.61: Q6.2 Q6.3 | C49.1 C47.1 26.12,41.45 | C52.- 10.52,69.95
  Top 1.016: 8.84,61.57 C51.- | R50.1 26.12,41.45 | U$2.5_R 88.85,66.75 | R56.2 3.93,85.08 v3.96,84.43
  Bottom 0.254: v72.24,62.33 v74.37,62.33 | v69.8,46.94 70.1,46.33 | v80.47,10.06 79.86,10.06 | v43.28,65.53 43.28,66.45
  Bottom 1.016: 88.85,66.75 88.54,66.45 | v3.96,84.43 3.96,84.12
  other vias: 72.39,69.49 84.58,11.73 90,11.25 90.76,13.75 87.5,13.75 85,13.75 82.5,13.75 80,13.75 77.5,13.75 76.25,15 75,13.75 91.25,8.75 92.5,12.5 90,2.5 91.25,2.5 92.5,2.5 92.5,3.75 93.75,3.75 93.75,2.5 95,3.75 95,5 97.5,2.5 98.75,2.5 80,17.5 82.5,17.5 87.9,16.28 88.75,20 88.75,22.5 86.25,22.5 83.75,22.5 82.5,21.25 91.25,20 91.25,22.5 93.75,22.5 98.75,25 80,30 82.5,31.25 83.75,31.25 93.75,31.25 92.5,26.25 90,26.25 90,28.75 95,30 80,32.5 85,35 82.5,35 80,35 82.5,37.5 80,40 80,37.5 78.75,37.5 76.25,36.25 75,36.25 73.75,36.25 90,45 90,42.5 92.5,42.5 90,40 92.5,40 90,37.5 87.5,37.5 85,40 87.5,40 87.5,45 85,47.5 83.75,48.75 82.5,50 81.25,51.25 80,52.5 78.75,53.75 77.5,53.75 75,53.75 75,50 71.25,50 73.75,47.5 72.5,45 75,45 76.25,43.75 80,43.75 81.25,42.5 83.75,41.25 72.5,53.75 70,53.75 67.5,53.75 65,53.75 63.75,51.25 63.75,48.75 97.5,56.25 97.5,55 97.5,52.5 97.5,50 95,48.75 92.5,48.75 85,55 85,52.5 92.5,52.5 95,52.5 82.5,55 77.5,56.25 78.75,56.25 85,56.25 85,60 87.5,60 90,60 92.5,57.5 95,57.5 97.5,60 97.5,62.5 95,65 92.5,62.5 90,62.5 85,62.5 87.5,62.5 82.5,62.5 80,62.5 78.75,60 85,65 87.5,65 87.5,67.5 90,50 90,52.5 87.5,50 87.5,52.5 76.25,56.25 73.75,56.25 71.25,56.25 71.83,57.68 68.75,56.25 66.25,56.25 63.75,56.25 63.75,60 63.75,61.25 67.5,61.25 66.25,61.25 65,61.25 87.5,72.5 88.75,73.75 86.25,73.75 97.5,68.75 97.5,72.5 96.25,77.5 96.25,80 97.5,81.25 97.5,83.75 95,75 95,72.5 91.25,73.75 88.75,76.25 87.5,82.5 86.25,82.5 86.25,85 91.25,86.25 92.5,86.25 92.5,83.75 91.25,83.75 98.75,86.25 98.75,88.75 98.75,91.25 98.75,93.75 98.75,96.25 98.75,98.75 96.25,98.75 82.5,98.75 77.5,98.75 78.75,97.5 81.25,97.5 77.5,95 77.5,90 77.5,92.5 77.5,87.5 75,98.75 71.25,97.5 67.5,98.75 71.25,87.5 70,90 75,92.5 75,90 72.5,92.5 72.5,90 70,85 75,85 72.5,85 67.5,85 70,82.35 72.5,82.35 70,80 67.5,77.5 67.5,80 67.5,82.35 60.21,82.35 62.5,77.5 61.25,73.75 60,75 58.75,76.25 57.2,77.8 57.5,82.5 60,97.5 57.5,95 57.5,97.5 55,97.5 55,95 62.5,95 65,95 67.5,92.5 68.75,93.75 62.5,91.25 53.75,85 53.75,82.5 53.75,80 53.75,77.5 53.75,75 55,70 57.5,70 57.5,67.5 58.75,65 57.5,62.5 58.75,60 57.5,57.5 58.75,55 57.5,52.5 75,77.5 77.5,77.5 80,75 50,70 47.5,70 40,70 38.75,76.25 47.5,76.25 47.5,80 45,80 42.5,80 42.5,87.5 42.5,85 42.5,82.5 47.5,82.5 45,82.5 45,85 47.5,87.5 47.5,85 47.5,90 45,90 42.5,90 37.5,98.75 36.25,98.75 35,98.75 33.75,98.75 20,97.5 20,95 20,92.5 21.25,92.5 22.5,90 25,87.5 22.5,87.5 20,87.5 20,90 15,92.5 13.75,90 12.5,97.5 12.5,95 12.5,92.5 10,97.5 10,95 1.25,97.5 5,95 5,92.5 3.75,88.75 1.25,95 1.25,92.5 1.25,87.5 1.25,85 7.5,85 7.5,78.75 8.75,77.5 1.25,77.5 1.25,80 7.5,67.5 7.5,65 7.5,60 5,60 12.5,73.75 60,16.25 60,13.75 57.5,16.25 57.5,13.75 55,16.25 55,13.75 52.5,16.25 52.5,13.75 50,13.75 47.5,13.75 42.5,12.5 45,12.5 56.25,10 56.25,8.75 55,10 38.75,7.5 36.25,7.5 32.5,5 30,5 27.5,3.87 25,3.87 25,1.25 17.5,2.5 15,2.5 11.25,3.75 8.75,3.75 11.25,1.25 8.75,1.25 3.75,1.25 1.25,1.25 20,12.5 22.5,12.5 25,12.5 27.5,12.5 17.5,16.25 18.75,20 18.75,21.25 20,20 20,18.75 21.25,17.5 7.5,27.5 10,27.5 12.5,27.5 3.75,37.5 20,35 28.75,36.25 28.75,37.5 30,36.25 28.75,35 27.5,33.75 28.75,38.75 38.75,65 41.25,65 28.75,65 33.75,67.5 32.5,66.25 31.25,65 30,66.25 31.25,67.5 28.75,67.5 33.75,71.25 31.25,71.25 30,72.5 32.5,72.5 31.25,75 28.75,83.75 30,81.25 15,48.75 15,50 11.25,51.25 20,52.5 11.25,57.5 17.5,56.25 23.75,52.5 11.25,63.75 43.75,17.5 39.51,13.23 46.25,17.5 47.5,17.5 48.75,17.5 50,18.75 53.75,22.5 52.5,23.75 52.5,22.5 56.25,20 57.5,20 53.75,27.5 57.5,26.25 52.5,35 51.25,35 48.75,33.75 46.25,38.75 45,38.75 8.57,19.24 11.43,21.22 14.94,21.98 48.78,4.67 76.74,7.2 74.36,20.7 88.23,93.69 89.57,91.74 14.36,19.54 36.83,53.42 58.17,45.04 60.15,45.34 70.82,35.13 33.78,50.06 41.4,50.37 41.25,48.39 40.64,52.05 79.76,25.31 91.43,5.79 72.38,76.52 78.93,69.51 70.25,66.47 69.03,67.84 69.79,71.49 65.37,72.1 51.81,74.09 95.09,33.85 95.7,35.99 96.31,38.42 96,42.39 65.22,13.43 68.57,22.57 72.84,25.32 31.08,44.52 62.84,45.85 60.17,47.91 50.4,78.32
  pour Bottom: 0,100 100,100 100,0 0,0
  pour Top: 0,100 100,100 100,0 0,0
GPS_EXTINT
  Top 0.254: GPS>.5 95.45,37.54 72.24,14.33 67.06,14.33 65.87,15.51 U2.36
GPS_NRESET
  Top 0.254: GPS>.6 97.08,40.08 71.93,14.94 67.21,14.94 66.37,15.77 U2.37
GPS_RXD
  Top 0.254: U2.51 84.58,28.49 87.17,31.09 96.01,39.93 96.01,41.15 97.48,42.62 GPS>.7
GPS_SCL
  Top 0.254: GPS>.3 92.2,32.46 72.85,13.11 66.75,13.11 64.87,14.98 U2.34
GPS_SDA
  Top 0.254: GPS>.4 93.83,35 72.54,13.72 66.9,13.72 65.37,15.25 U2.35
GPS_TXD
  Top 0.254: U2.52 84.16,28.99 86.56,31.39 95.4,40.23 95.4,42.67 97.89,45.16 GPS>.8
IND_LED_B
  Top 0.254: U2.26 51.22,30.49 49.68,28.96 49.38,28.65 49.38,24.38 49.38,22.25 47.24,20.12 47.09,19.96 41.76,19.96 39.32,17.53 39.32,16.12 R11.2
IND_LED_G
  Top 0.254: U2.25 51.11,30.99 49.07,28.96 48.92,28.8 48.92,24.38 48.92,22.4 46.94,20.42 41.49,20.42 R10.2
IND_LED_R
  Top 0.254: U2.28 51.44,29.49 50.29,28.35 50.29,24.38 50.29,22.1 50.29,21.95 47.4,19.05 42.22,19.05 40.39,17.22 40.39,12.92 R15.2
IND_LED_W
  Top 0.254: U2.27 51.33,29.99 49.99,28.65 49.84,28.5 49.84,24.38 49.84,22.1 47.55,19.81 47.24,19.51 42.06,19.51 39.93,17.37 39.93,14.6 R14.2
INT_POWER  (via drill 0.3)  (1 unrouted)
  Top 0.15: L3.2 85.58,67.77 C30.1 | C29.2 80.33,69.44
  Top 0.254: C23.2 C27.2 71.89,65.88 IC4.17 71.89,65.64 71.63,65.38 69.34,65.38 69.19,65.53 v69.19,66.75 | C26.2 C22.2 | C25.2 C21.2 | 85.34,69.1 C30.1 | L3.2 85.48,67.35 | C25.2 77.79,66.08 78.64,65.23 83.21,65.23 85.34,67.36 | 77.57,72.69 C26.2 | IC4.1 76.13,68.49 v76.81,67.82 77.57,67.06 C25.2 | v76.81,70.41 76.39,69.99 IC4.4 | 80.33,69.44 79.86,69.92 79.86,70.1 79.55,70.41 v76.81,70.41 | L2.1 80.38,67.72 C29.2 | v76.81,70.41 76.81,71.02 77.57,71.78 C26.2
  Bottom 0.254: v76.81,70.41 v76.81,67.82 76.2,67.21 69.65,67.21 v69.19,66.75
MCU_WAKEUP  (via drill 0.3)
  Top 0.254: D9.C D8.C D2.C D3.C D4.C D5.C 41.93,6.84 40.84,7.92 40.84,17.07 42.37,18.59 47.55,18.59 50.9,21.95 50.9,28.35 51.21,28.65 v58.67,28.65 | U2.14 65.37,39.17 62.79,41.76 v58.22,41.76
  Bottom 0.254: v58.67,28.65 59.13,29.11 59.13,41.45 58.83,41.76 v58.22,41.76
N$1
  Top 0.254: LED2.A R10.1
N$2
  Top 0.254: C12.2 98.23,6.62 96.93,7.92 96.81,7.92 R6.1
N$3  (via drill 0.3)
  Top 0.254: LED1.C v33.07,88.39 | v52.73,88.39 52.66,88.32 IC2.30
  Bottom 0.254: v33.07,88.39 v52.73,88.39
N$4
  Top 0.254: LED3.A R11.1
N$5
  Top 0.254: Q1.1 76.29,51.82 66.75,51.82 65.53,50.6 65.6,50.53 C15.1 65.5,48.52 R9.1
N$6
  Top 0.254: U2.5 69.87,37.87 71.32,39.32 71.32,48.53 C14.1 74.83,48.62 78.64,44.81 83.3,44.81 Q1.2
N$7
  Top 0.254: R5.1 84.85,8.42 86.41,6.86 86.63,6.86 C13.2
N$8
  Top 0.254: R23.2 26.94,8.99 LED11.A
N$9
  Top 0.254: R9.2 67.55,46.02 69.8,46.02 70.87,44.96 70.87,40.08 70.87,39.47 70.1,38.71 69.37,37.98 U2.6
N$10
  Top 0.254: U3.3 21.13,6.6 22.25,5.49 22.38,5.35 C19.3
N$11
  Top 0.254: R12.1 73.8,7.32 74.07,7.32 74.61,6.77 C17.2
N$12
  Top 0.254: LED4.A R14.1
N$13
  Top 0.254: LED9.A R21.2
N$15
  Top 0.254: U3.2 18.65,5.94 19.66,5.94 19.98,5.62 C19.1
N$16
  Top 0.254: LED5.A R15.1
N$17
  Top 0.254: J1.D- 4.9,7.62 6.1,7.62 7.11,6.6 U3.18
N$18
  Top 0.254: C18.2 62.85,7.32 62.64,7.32 61.38,8.57 R16.1
N$19
  Top 0.254: LED6.A R18.2
N$20
  Top 0.254: J1.D+ 6.1,7.01 7.15,5.95 U3.19
N$21
  Top 0.254: 9.08,9.45 C20.1 9.45,9.08 9.45,8.23 10.42,7.25 U3.17
N$22
  Top 0.254: LED7.A R19.2
N$23
  Top 0.254: R24.2 26.94,7.32 LED12.A
N$24
  Top 0.254: LED10.A R22.2
N$25
  Top 0.254: LED8.A R20.2
N$26
  Top 0.254: 23.05,8.86 LED11.C 22.75,8.55 U3.6
N$27
  Top 0.254: U3.5 18.66,7.92 21.34,7.92 22.57,7.92 LED12.C
N$28
  Top 1.016: Q3.3 19.46,24.69 D1.A 22.2,21.95 JP2.2
N$29
  Top 0.254: J2.SHIELD1 J2.SHIELD3 J2.SHIELD2 4.48,14.54 FB4.2
N$30
  Top 0.254: J2.GND 4.93,19.2 5.79,19.2 6.4,18.59 FB3.2
N$31
  Top 0.254: J2.VBUS 5.87,21.87 6.86,22.86 FB1.1
N$32
  Top 0.254: J2.ID 4.9,19.96 5.94,19.96 8.35,17.56 R26.1 10.34,19.36 U4.4 10.01,20.07
N$33
  Top 0.254: IC4.19 72.89,61.77 69.49,58.37 Q4.2
N$34
  Top 0.254: IC4.20 73.39,58.89 73.61,58.67 | 73.15,58.67 73.61,58.67 | 73.61,58.67 74.93,58.67 Q4.1
N$35
  Top 0.254: Q2.E 12.8,16.83 R27.1
N$36
  Top 0.254: R28.1 11.28,14.9 Q2.B R29.2
N$37
  Top 0.254: RF_SYSCLK.TP 34.44,35.05 46.02,35.05 58.83,47.85 58.83,49.99 59.44,50.6 59.44,67.06 63.7,71.32 66.75,71.32 69.95,74.52 71.63,74.52 72.89,73.26 IC4.7
N$38
  Top 0.254: U5.15 37.05,59.27 R62.1 38.44,60.77 36.88,62.33 36.76,62.33 R35.2
N$39
  Top 0.254: L4.1 83.97,74.89 C28.1
N$40
  Top 0.254: 81.84,74.89 C31.1 81.99,73.29 L1.1
N$42
  Top 0.254: L6.1 81.93,83.01 C34.2 C32.2 81.93,76.99 C31.2
N$43
  Top 0.254: C35.2 83.99,83.11 L5.2 83.88,80.97 C33.1 84.12,78.86 C28.2
N$45
  Top 0.254: 83.92,84.87 C35.1 | L7.1 84.04,88.78 C36.2 83.97,86.96 C35.1 | L6.2 82.04,84.82 C35.1
N$46
  Top 0.254: R41.2 47.97,65.11 48.01,65.08 | D6.C 44.31,65.75 D7.C 44.99,65.08 46.94,65.08 | R42.1 46.94,65.08 | 46.94,65.08 48.01,65.08 | 48.01,65.08 48.72,65.08 Q6.4
N$47
  Top 0.254: BAT.2 35.2,39.42 35.2,41.87 R31.1
N$48
  Top 0.254: BAT.3 R32.1
N$49
  Top 0.254: BAT.4 40.39,39.42 R33.1
N$50
  Top 0.254: R33.2 39.23,45.08 C39.1 38.86,46.55 38.86,49.53 38.25,50.14 37.7,50.69 U5.7
N$51
  Top 0.254: U5.6 37.05,49.27 C40.1 37.64,48.09 37.64,44.08 R32.2
N$52
  Top 0.254: 35.81,48.09 C41.1 | U5.5 36.4,49.27 C41.1 | R31.2 35.36,48.23 C41.1
N$53
  Top 0.254: R30.2 34.23,45.23 C38.1 34.59,46.4 34.59,47.09 34.59,49.53 35.75,50.69 U5.4 U5.3
N$54
  Top 0.254: U5.1 33.8,52 33.29,52 R34.2 32.16,51.24 32.16,55.39 C43.1
N$55
  Top 0.254: R36.1 48.83,45.89 R38.2
  Top 0.61: Q5.1 Q5.2 Q5.3
  Top 0.813: Q5.3 51.69,48.31 51.69,45.84 | 51.69,45.84 R36.1 | R39.2 52.14,46.29 51.69,45.84
N$56  (via drill 0.3)
  Top 0.254: C42.2 34.75,59.44 35.81,58.37 35.81,57.57 U5.17 35.75,55.99 v35.81,55.93 | v34.59,53.49 34.45,53.35 U5.2
  Bottom 0.254: v35.81,55.93 35.81,54.71 v34.59,53.49
N$57
  Top 0.254: R38.1 46.99,48.04 C45.2 47.24,48.53 C46.1 46.24,51.21 40.54,51.21 40.14,51.61 U5.10 39.65,51.21
N$58
  Top 0.254: 45.17,49.99 C44.2 45.02,49.99 C45.1 43.09,48.16 R37.1 42.79,48.04 41.15,49.68 40.08,49.68 39,50.76 U5.9
N$59
  Top 1.016: Q5.8 Q5.7 51.05,55.66 | 51.05,55.66 Q5.6 Q5.5 | Q6.5 Q6.6 Q6.7 Q6.8 51.05,59.09 51.05,55.66
N$60
  Top 0.254: U5.16 36.42,57.53 R35.1
N$61
  Top 0.61: 16.78,59.91 C63.+ | L8.2 21.64,55.33 21.64,55.17 21.64,50.29 19.2,47.85 14.63,47.85 13.31,46.53 IC1.5
  Top 1.016: L8.2 16.78,59.91
N$62  (via drill 0.3)
  Top 0.254: R40.1 v47.4,54.71 | v54.56,54.71 55.32,53.95 55.32,50.02 R39.1 53.49,49.58 Q5.4
  Bottom 0.254: v47.4,54.71 v54.56,54.71
N$63
  Top 0.254: U5.11 39.65,56.63 R40.2
N$64
  Top 0.254: R43.2 44.72,62.67 D7.A 44.96,61.42 45.6,60.77 R42.2
N$65
  Top 0.254: U5.13 38.35,58.62 38.56,58.83 40.88,58.83 R43.1
N$66
  Top 0.254: U5.14 37.7,58.73 38.25,59.28 39.47,59.28 40.39,60.2 40.39,60.47 R44.1
N$69
  Top 0.406: J4.VBUS 4.78,32.92 5.49,32.92 5.79,33.22
  Top 0.61: L8.1 23.2,62.79 14.63,62.79 8.53,56.69 8.53,51.82 11.12,49.23 11.12,49.07 | 5.79,33.22 11.28,33.22 13.11,35.05 14.12,35.05 C48.+ 13.41,35.36 9.14,39.62 9.14,47.09 11.12,49.07 | 11.12,49.07 IC1.7
N$70
  Top 0.406: R49.2 26.1,47.74 26.16,47.81
  Top 0.61: 26.08,50.43 L8.4 26.16,50.81 26.16,47.81 | 26.52,49.99 25.6,49.99
  Top 1.016: 26.08,50.43 26.52,49.99 | 25.6,49.99 25.3,50.29 | 26.16,47.81 R50.2
N$71
  Top 0.254: R45.2 C47.2
N$72
  Top 0.254: R45.1 IC1.1
N$73
  Top 0.254: R46.1 Q7.3
N$74  (via drill 0.3)
  Top 0.254: 16.76,46.02 v16.8,45.99 R48.1 | R47.2 R46.2 23.66,29.38 v23.47,29.57
  Bottom 0.254: v23.47,29.57 23.47,37.49 23.93,37.95 23.93,40.08 17.98,46.02 16.84,46.02 v16.8,45.99
N$76
  Top 0.254: R48.2 14.9,43.99 IC1.3
  Top 0.406: 19.36,44.65 19.36,44.43 C49.2 18.93,44.08 18.93,45.84 | R49.1 18.93,45.84 | 18.93,45.84 17.98,46.79 15.7,46.79 14.94,46.02 14.94,44.08 R48.2
N$77  (via drill 0.3)
  Top 0.406: v1.52,39.93 R51.1 | R52.2 v22.25,39.17
  Bottom 0.406: v1.52,39.93 4.32,42.72 IC1.2 10.16,39.17 v22.25,39.17
N$78
  Top 0.254: B4.2 31.92,85.95 31.92,93.15 29.72,95.35 CONFIG_INTERFACE_TEST_POINT.2
N$80
  Top 0.254: R3.1 36.56,90.27 LED1.A 36.56,86.76 B3.2 | R3.1 36.46,94.05 U1.3 | IC2.4 38.1,90.52 37.95,90.37 R3.1
N$81
  Top 1.016: JP2.1 24.74,21.95 D1.C 28.19,23.36 B5.2
N$82
  Top 0.254: B6.2 C24.2 67.06,66.75 67.97,67.67 68.8,68.49 69.63,68.49 IC4.15
N$83
  Top 0.61: U$2.3 94.91,76.14 B7.2
N$84  (via drill 0.3)
  Top 0.254: R60.2 4,81.65 5.49,80.16
  Top 0.406: C53.+ 67.21,95.4 65,93.19 IC3.2
  Top 0.61: 7.47,88.24 IC5.2 | JP3.2 4.06,78.74 5.49,80.16 10.06,84.74 | v63.7,92.2 IC3.2
  Top 1.016: C56.+ 7.47,88.24 | 10.06,84.74 IC5.2
  Bottom 0.61: JP3.2 4.06,78.74 5.64,80.31 28.8,80.31 35.97,73.15 53.95,73.15 63.7,82.91 v63.7,92.2
N$85
  Top 0.254: R54.1 64.92,97.23 70.26,97.23 71.63,95.86 71.63,94.03 67.51,89.92 R53.2 66.6,89.92 66.6,87.64
  Top 0.61: C55.+ 67.56,87.64 66.6,87.64 IC3.1
N$86
  Top 0.254: C11.2 R59.1
N$87
  Top 0.305: J4.ID 17.87,30.9 USB_ID.TP
N$88
  Top 0.305: J4.D+ 17.22,31.55 USB_DP.TP
N$89
  Top 0.254: IC5.1 14.33,85.8 14.33,86.11 13.41,87.17 R55.2 12.5,88.7 8.99,92.2 7.01,92.2 5.79,90.98 R56.1 5.79,86.26
  Top 0.61: C58.+ 16,86.87 IC5.1
N$90
  Top 0.305: J4.D- 15.59,32.2 USB_DN.TP
N$91
  Top 0.61: L8.3 14.01,53.95
  Top 1.016: D10.A 10.71,53.94 | 10.67,54.86 10.67,53.84 D10.A | 14.01,53.95 C63.- 13.41,53.95 13.26,53.8 D10.A
N$92
  Top 0.254: IC6.1 26.52,71.78 26.67,71.78 27.58,72.69 R57.2 27.89,73.61 31.39,77.11 31.39,79.1 30.48,80.01 26.36,80.01 R58.1
  Top 1.016: C61.+ 27.74,69.49 IC6.1
NRST  (via drill 0.3)  (1 unrouted)
  Top 0.254: R4.2 40.09,4.7 S1.P$4 42.67,4.66 42.67,3.2 | 42.67,3.2 33.98,3.2 BTN_NRST.TP 33.68,2.1 R59.2 | 42.67,3.2 v50.75,3.2 50.75,1.81 S1.P$3 | U2.7 68.89,36.98 v68.89,35.36 | v72.54,40.54 73.15,41.15 74.37,41.15 | 74.37,41.15 81.38,41.15 v87.78,34.75 | 74.37,41.15 74.37,42.82 NRST_MCU.TP
  Bottom 0.254: v68.89,35.36 72.54,39.01 v72.54,40.54 | v50.75,3.2 60.2,3.2 61.57,1.83 65.84,1.83 67.06,3.05 78.44,3.05 PR0>.5 | 97.99,24.23 89.09,33.14 89.09,33.44 v87.78,34.75
POW_LED_G1
  Top 0.254: U2.22 50.78,32.49 49.99,31.7 47.55,29.26 47.55,27.74 46.21,26.4 R20.1
POW_LED_G2
  Top 0.254: U2.21 50.67,32.99 49.68,32 47.55,29.87 46.21,28.53 R19.1
POW_LED_G3
  Top 0.254: U2.20 50.56,33.49 49.38,32.31 47.7,30.63 R18.1
POW_LED_R
  Top 0.254: U2.24 51,31.49 50.6,31.09 48.46,28.96 48.46,24.2 R21.1
POW_LED_Y
  Top 0.254: U2.23 50.89,31.99 50.29,31.39 48.01,29.11 48.01,26.52 48.01,25.87 R22.1
RF_SIGNAL
  Top 0.254: C37.2 84.04,92.42 | RF_SIGNAL.TP 88.85,88.84 U$2.1 94.64,91.52 94.64,94.18 93.12,95.71 85.5,95.71 84.04,94.25 C37.2 | L7.2 84.04,90.6 C37.2
RF_SIGNAL_AMPLIFIED
  Top 0.61: J3.S 95.25,55.78 98.6,59.13 98.6,64.41 U$2.4
SPI2_CLK  (via drill 0.3)
  Top 0.254: v60.35,49.07 60.66,49.38 60.66,67.06 64.01,70.41 67.06,70.41 70.26,73.61 71.32,73.61 71.89,73.04 IC4.9 | v60.05,28.65 60.39,28.99 U2.29 | SPI2_CLK.TP 32.61,19.51 35.05,21.95 35.05,28.65 39.01,32.61 46.63,32.61 55.78,41.76 v56.69,41.76
  Bottom 0.254: v60.35,49.07 59.13,47.85 59.13,44.2 v56.69,41.76 56.69,28.65 58.52,26.82 59.44,26.82 60.05,27.43 v60.05,28.65
SPI2_IRQ  (via drill 0.3)  (1 unrouted)
  Top 0.254: v69.49,44.81 70.41,43.89 70.41,39.93 68.43,37.95 68.43,37.05 | SPI2_IRQ.TP 32,22.86 34.44,25.3 34.44,28.8 38.71,33.07 46.48,33.07 55.78,42.37 62.79,42.37 63.7,43.28 v63.7,45.11 63.7,46.33 62.48,47.55 62.48,66.9 64.58,68.99 IC4.14
  Bottom 0.254: v63.7,45.11 69.19,45.11 v69.49,44.81
SPI2_MISO  (via drill 0.3)
  Top 0.254: U2.10 67.37,38.72 v67.97,39.32 | v60.96,47.85 61.27,48.16 61.27,67.06 64.16,69.95 67.21,69.95 70.41,73.15 71.17,73.15 71.39,72.93 IC4.10 71.39,71.71 | SPI2_MISO.TP 32.46,28.35 38.1,33.98 46.18,33.98 56.39,44.2 v60.96,44.2
  Bottom 0.254: v67.97,39.32 65.23,39.32 60.96,43.59 v60.96,44.2 v60.96,47.85
SPI2_MOSI  (via drill 0.3)
  Top 0.254: v61.87,46.63 61.87,67.06 64.31,69.49 67.36,69.49 67.86,69.99 IC4.12 | U2.11 66.9,37.02 66.9,39.32 68.89,41.3 v68.89,41.76 | SPI2_MOSI.TP 32.61,25.3 33.83,26.52 33.83,28.96 38.41,33.53 46.33,33.53 56.24,43.43 v62.64,43.43
  Bottom 0.254: v68.89,41.76 68.58,42.06 64.01,42.06 v62.64,43.43 61.87,44.2 v61.87,46.63
SPI2_SEL_RFTX  (via drill 0.3)
  Top 0.254: v69.19,43.28 69.95,42.52 69.95,40.08 67.87,38 U2.9 | 59.44,47.85 59.44,49.68 60.05,50.29 60.05,67.06 63.86,70.87 66.9,70.87 70.1,74.07 71.48,74.07 72.39,73.15 IC4.8 | SPI2_SEL_RFTX.TP 32,31.39 34.75,31.39 37.95,34.59 46.18,34.59 59.44,47.85 | v62.64,44.5 59.44,47.7 59.44,47.85
  Bottom 0.254: v69.19,43.28 64.01,43.28 62.79,44.5 v62.64,44.5
SWD_RXD
  Top 0.254: U2.16 64.37,38.65 62.48,40.54 60.05,40.54 57,37.49 55.17,35.66 55.02,35.66 SWD_RXD.TP
SWD_TXD
  Top 0.254: U2.17 62.73,34.99 63.4,35.66 63.4,39.01 62.48,39.93 62.18,39.93 60.35,39.93 60.05,39.62 57.91,37.49 SWD_TXD.TP
SWDCLK  (via drill 0.3)
  Top 0.254: U2.49 76.75,27.49 78.64,25.6 v78.64,23.16 | PR0>.3 84.28,17.53 v81.99,19.81
  Bottom 0.254: v81.99,19.81 v78.64,23.16
SWDIO  (via drill 0.3)
  Top 0.254: U2.46 70.87,22.7 70.87,22.09 v73.15,19.81 | v77.11,15.85 77.98,14.99 PR0>.2
  Bottom 0.254: v73.15,19.81 76.81,16.15 v77.11,15.85
USB_DATA_N  (via drill 0.3)
  Top 0.254: U4.1 8.57,21.22 7.01,21.22 | 7.01,21.22 J2.D- | U2.44 69.87,27.07 69.41,27.54 65.53,27.54 v65.53,27.15 | v59.57,24.25 59.27,24.55 50.07,15.34 42.06,15.34 v42.06,14.96 | v7.01,21.95 7.01,21.22
  Bottom 0.254: v65.53,27.15 65.53,27.54 62.26,27.54 59.27,24.55 v59.57,24.25 | v42.06,14.96 42.06,15.34 20.64,15.34 14.04,21.95 v7.01,21.95
USB_DATA_P  (via drill 0.3)
  Top 0.254: U2.45 70.37,27.14 69.58,27.94 65.53,27.94 v65.53,28.32 | v58.69,25.13 58.99,24.83 49.9,15.75 42.06,15.75 v42.06,16.13 | v15.48,21.32 15.32,21.23 14.55,20.46 R27.2 12.69,20.57 U4.2 J2.D+
  Bottom 0.254: v65.53,28.32 65.53,27.94 62.1,27.94 58.99,24.83 v58.69,25.13 | v42.06,16.13 42.06,15.75 20.81,15.75 15.32,21.23 v15.48,21.32
V+STM
  Top 0.254: C9.1 78.39,34.68 C8.1 76.04,34.99 U2.64 73.52,34.99 72.85,35.66 | C10.2 C5.2 65.87,41.02 U2.13 65.87,36.23 66.14,35.97 67.06,35.97 67.82,35.2 67.82,33.99 | C4.1 74.13,39.01 72.85,39.01 71.87,38.04 U2.1 71.93,36.93 71.93,36.58 72.69,35.81 72.85,35.66 | 61.57,27.13 61.93,27.49 U2.32 63.46,27.49 66.75,30.79 67.67,31.7 67.67,33.99 | 61.57,27.13 61.57,25.54 C6.2 | 61.57,27.13 61.57,25.6 61.87,25.3 62.03,25.3 62.79,24.54 62.94,24.38 63.09,24.23 63.09,22.32 B1.2 | C16.2 61.35,38.8 60.35,37.8 60.2,37.64 60.2,34.9 61.11,33.98 U2.19 67.67,33.99 | 67.67,33.99 67.82,33.99 | 67.82,33.99 71.18,33.99 72.85,35.66
VIBRATOR  (via drill 0.3)
  Top 0.254: R25.1 Q3.1 16.24,26.82 v17.37,26.82 | v78.64,27.13 78.64,27.43 78.03,28.04 73.92,28.04 U2.50
  Bottom 0.254: v17.37,26.82 18.29,27.74 25.3,27.74 30.48,32.92 45.72,32.92 59.74,18.9 70.71,18.9 78.64,26.82 v78.64,27.13

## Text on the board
Top: WPLB / Main / V1_0
tNames: Charge | Native | NRST / 3V3 / SWDCLK / SWDIO / GND | FTDI
bNames: WatchPLB Mainboard V1.0 / c by Samuel Hick, HSD 2018 / Made in Austria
